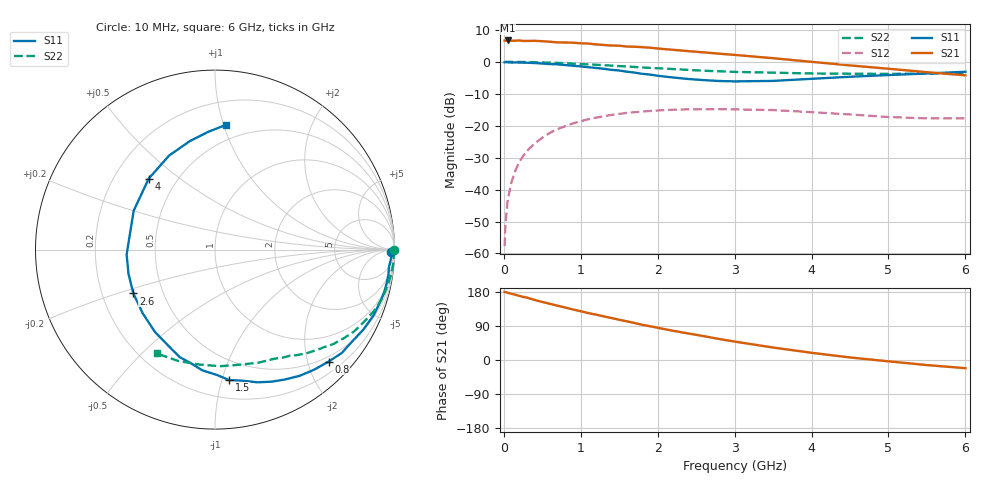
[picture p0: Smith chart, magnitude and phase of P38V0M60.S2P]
! SIEMENS Small Signal Semiconductors
! BFP181
! Si NPN RF Bipolar Junction Transistor in SOT143
! VCE = 8 V  IC = 0.6 mA
! Common Emitter S-Parameters:  March  1996
# GHz  S  MA  R  50
!  f  S11  S21  S12  S22
! GHz  MAG  ANG  MAG  ANG  MAG  ANG  MAG  ANG
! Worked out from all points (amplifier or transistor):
!   36 points, 10 MHz to 6 GHz, reference 50 ohm
!   highest |S21| = 6.7 dB at 50 MHz (marker M1)
!   |S21| within 3 dB of that: start of sweep to 2.233 GHz
!   unconditionally stable (mu >= 1): 3.736 GHz to end of sweep
!   at 250 MHz: K = 0.08, MSG = 18.0 dB, |S12| = -29.5 dB
!   at 1.4 GHz: K = 0.43, MSG = 10.9 dB, |S12| = -16.6 dB
!   at 6 GHz: K = 1.38, MAG = 3.1 dB, |S12| = -17.7 dB
!   S11 on the Smith chart (normalised r, x): 10 MHz: 73, -45; 800 MHz: 0.40, -2.38; 1.5 GHz: 0.34, -1.05; 2.6 GHz: 0.34, -0.22; 4 GHz: 0.35, +0.39; 6 GHz: 0.38, +1.02
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0.01  0.9803 -0.7  2.147 179.7  0.0013 74.2  0.9989 -0.2
0.02  0.9827 -1.2  2.129 179.5  0.0027 85.9  0.9979 -0.6
0.05  0.9821 -2.8  2.157 177.4  0.0069 92.1  0.9971 -1.4
0.1  0.9742 -5.7  2.133 174.8  0.0131 85.1  0.9962 -2.8
0.15  0.9764 -8.3  2.135 172.1  0.0198 83.3  0.9955 -4.1
0.2  0.9743 -11.3  2.154 169.3  0.0269 82.5  0.9948 -5.5
0.3  0.9674 -16.8  2.119 164.6  0.0401 78.1  0.99 -8.2
0.4  0.956 -22.6  2.129 158.5  0.0527 74.5  0.9844 -10.9
0.5  0.9392 -28.3  2.099 153.1  0.0648 70.1  0.9769 -13.6
0.8  0.8886 -44.6  2.005 138.3  0.0984 58.8  0.9494 -21.1
0.9  0.8675 -50.5  1.988 133.3  0.1087 55.0  0.9348 -23.6
1.1  0.822 -61.7  1.928 123.7  0.1264 48.1  0.91 -28.2
1.5  0.7306 -83.9  1.785 106.2  0.1526 35.8  0.8566 -36.4
1.9  0.6307 -108.1  1.662 89.1  0.1698 25.0  0.8025 -43.7
2.2  0.568 -126.0  1.539 77.1  0.1778 18.0  0.7695 -48.7
2.6  0.5164 -151.8  1.404 62.9  0.1807 9.9  0.7237 -54.8
3  0.4932 -176.8  1.282 48.6  0.18 2.1  0.6942 -60.9
3.5  0.5022 154.4  1.138 32.9  0.1755 -5.3  0.6758 -68.6
4  0.5412 133.0  0.998 19.0  0.1628 -10.8  0.6564 -77.6
4.5  0.583 116.0  0.878 6.7  0.1498 -14.4  0.6503 -87.6
5.5  0.6563 93.5  0.687 -13.4  0.1301 -11.6  0.6535 -108.4
6  0.6975 85.0  0.614 -21.6  0.1303 -8.4  0.6634 -119.3
